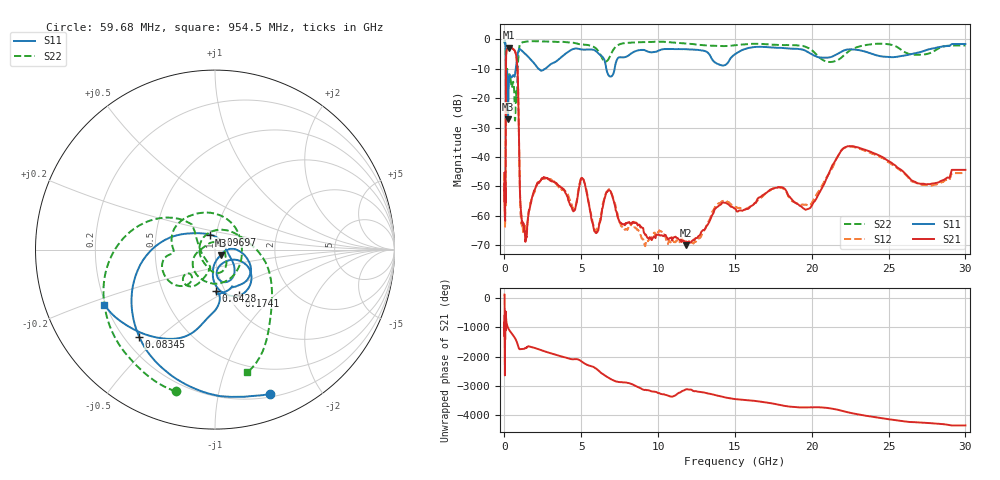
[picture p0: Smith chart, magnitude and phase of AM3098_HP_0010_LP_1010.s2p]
! Date/Time: Thu, Feb 28, 2019 8:33 AM
! Network Analyzer: Agilent Technologies E8364B Rev: A.07.50.67
! Sweep from 0.010 to 30.000 GHz, 1601 Points, Sweep Type: LOG
! Power Supply: 5.022 V, 0.002 A
# Hz S DB R 50
!freq MagS11 AngS11 MagS21 AngS21 MagS12 AngS12 MagS22 AngS22
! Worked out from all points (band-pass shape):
!   1601 points, 10 MHz to 30 GHz, reference 50 ohm
!   highest |S21| = -2.79 dB at 267.8 MHz (marker M1); lowest = -69.9 dB at 11.83 GHz (marker M2)
!   |S21| within 3 dB of the highest: 107.2 MHz to 772.1 MHz (664.9 MHz wide, 151 % of centre)
!   lowest |S11| = -27.2 dB at 233.9 MHz (marker M3), VSWR 1.09, Z = 53.3 - j3.12 ohm
!   |S11| at or under -10 dB: 92.11 MHz to 730.5 MHz (638.4 MHz wide, 155 % of centre); 2.225 GHz to 2.648 GHz (423.6 MHz wide, 17.4 % of centre); 6.63 GHz to 7.17 GHz (540.6 MHz wide, 7.83 % of centre)
!   |S22| runs from -27.6 to -0.6 dB; largest |S21 - S12| = 0.01
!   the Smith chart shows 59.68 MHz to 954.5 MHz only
!   S11 on the Smith chart (normalised r, x): 59.68 MHz: 0.23, -1.42; 83.45 MHz: 0.26, -0.43; 96.97 MHz: 0.93, +0.16; 174.1 MHz: 1.12, -0.63; 642.8 MHz: 0.91, -0.45; 954.5 MHz: 0.19, -0.23
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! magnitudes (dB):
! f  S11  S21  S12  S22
! 10 MHz  -0.3  -45.4  -45.9  -0.6
! 38.04 MHz  -0.5  -59.2  -63.1  -1.0
! 59.68 MHz  -1.3  -53.7  -51.9  -1.7
! 83.45 MHz  -3.8  -34.0  -33.8  -4.3
! 96.97 MHz  -21.0  -10.1  -10.1  -22.2
! 144.7 MHz  -15.1  -3.5  -3.5  -13.0
! 174.1 MHz  -10.8  -3.3  -3.3  -10.0
! 233.9 MHz  -27.2  -2.9  -2.8  -12.4
! 267.8 MHz  -17.3  -2.8  -2.8  -12.7
! 550.5 MHz  -12.2  -3.3  -3.2  -14.5
! 642.8 MHz  -12.7  -3.6  -3.6  -18.8
! 842.3 MHz  -5.6  -9.8  -9.8  -13.6
! 954.5 MHz  -3.3  -37.3  -37.3  -3.0
! 1.087 GHz  -3.6  -59.0  -61.7  -1.2
! 1.382 GHz  -5.0  -68.3  -65.2  -0.7
! 2.084 GHz  -9.2  -49.6  -49.9  -0.6
! 5.077 GHz  -3.4  -47.3  -47.0  -1.7
! 7.926 GHz  -5.9  -62.7  -64.5  -1.2
! 11.83 GHz  -3.3  -69.9  -69.0  -1.4
! 19.7 GHz  -4.2  -57.8  -56.4  -2.7
! 22.56 GHz  -3.4  -36.3  -36.5  -3.5
! 30 GHz  -1.6  -44.4  -45.5  -2.0
